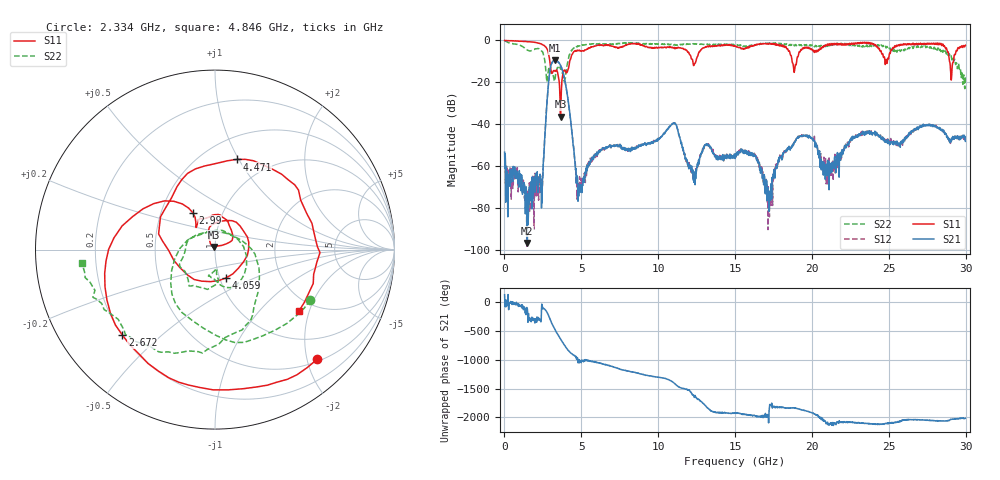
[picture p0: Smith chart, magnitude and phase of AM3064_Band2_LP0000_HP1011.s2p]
# Hz S DB R 50.0
!freq dBS11 angS11 dBS21 angS21 dBS12 angS12 dBS22 angS22
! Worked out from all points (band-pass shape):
!   1600 points, 10 MHz to 29.98 GHz, reference 50 ohm
!   highest |S21| = -9.45 dB at 3.29 GHz (marker M1); lowest = -96.9 dB at 1.491 GHz (marker M2)
!   |S21| within 3 dB of the highest: 3.009 GHz to 3.673 GHz (664.2 MHz wide, 19.9 % of centre)
!   lowest |S11| = -36.4 dB at 3.646 GHz (marker M3), VSWR 1.03, Z = 49.5 + j1.4 ohm
!   |S11| at or under -10 dB: 2.951 GHz to 4.24 GHz (1.289 GHz wide, 35.8 % of centre); 18.71 GHz to 19.01 GHz (296.2 MHz wide, 1.57 % of centre); 28.95 GHz to 29.2 GHz (257.2 MHz wide, 0.884 % of centre)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
!   |S22| runs from -23.1 to -0.2 dB; largest |S21 - S12| = 0.011
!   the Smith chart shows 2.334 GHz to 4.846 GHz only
!   S11 on the Smith chart (normalised r, x): 2.334 GHz: 0.54, -2.18; 2.672 GHz: 0.20, -0.38; 2.99 GHz: 0.72, +0.32; 4.059 GHz: 1.07, -0.35; 4.471 GHz: 0.71, +0.98; 4.846 GHz: 1.66, -1.71
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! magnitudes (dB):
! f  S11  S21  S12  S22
! 10 MHz  0.0  -53.4  -61.2  -0.2
! 1.491 GHz  -0.6  -96.9  -78.5  -4.7
! 2.334 GHz  -1.6  -64.7  -72.6  -4.4
! 2.672 GHz  -3.1  -40.1  -40.1  -12.8
! 2.99 GHz  -12.4  -13.1  -13.1  -14.3
! 3.29 GHz  -14.8  -9.4  -9.6  -18.4
! 3.646 GHz  -36.4  -11.8  -12.0  -13.7
! 4.059 GHz  -15.4  -24.5  -24.4  -12.3
! 4.471 GHz  -5.7  -50.4  -49.8  -3.8
! 4.846 GHz  -4.7  -71.0  -70.9  -2.6
! 5.015 GHz  -5.1  -69.3  -69.0  -2.5
! 10 GHz  -3.4  -47.6  -47.7  -1.7
! 11.09 GHz  -4.0  -39.5  -39.7  -2.0
! 12.34 GHz  -11.4  -66.3  -65.9  -1.6
! 13.13 GHz  -3.2  -49.6  -49.6  -2.1
! 15 GHz  -2.6  -56.5  -55.4  -1.9
! 17.25 GHz  -1.5  -72.7  -73.1  -1.2
! 18.04 GHz  -2.5  -57.2  -54.9  -1.9
! 19.99 GHz  -4.2  -46.9  -46.8  -2.1
! 21.02 GHz  -1.8  -57.5  -68.6  -2.5
! 25 GHz  -8.4  -48.9  -48.0  -3.2
! 29.98 GHz  -2.3  -48.2  -47.7  -17.3
